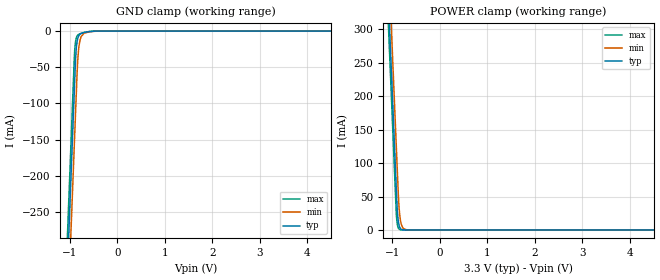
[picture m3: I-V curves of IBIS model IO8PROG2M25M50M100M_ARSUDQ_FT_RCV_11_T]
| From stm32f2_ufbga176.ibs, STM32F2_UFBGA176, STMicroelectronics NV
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| *** New cell (Generated with 5.14beta1 (Sep 20 2010 13:23:23))
[Model]   IO8PROG2M25M50M100M_ARSUDQ_FT_RCV_11_T
Model_type Input
Polarity   Non-Inverting
Enable   Active-Low
| CAP_THRESHOLD on pad IOV33 is "CMOS" :
| Rising=10.0% of vddio   Falling=90.0% of vddio
| C_comp min and max val. don't necessarily correlate with the min and max pvt
| but are the smallest and greatest pad capacitance found.
| var   typ   min   max
C_comp   2.14000pF  2.04120pF  2.26005pF
Vinl = 800.0mV | Dummy value overriden by next lines
Vinh = 2.00V | Dummy value overriden by next lines
[Model Spec]
| TIME_THRESHOLD on pin ZIV33 is "CORE" :
| Rising=40.0% of vddio   Falling=60.0% of vddio
Vinl 1.48450V 1.23350V 1.61250V
Vinh 1.48450V 1.23350V 1.61250V
| variable   typ   min   max
[Temperature Range] 25.0 125.0 -40.0
| variable   typ   min   max
[Voltage Range] 3.3V 2.7V 3.6V
| variable   typ   min   max
[POWER Clamp Reference] 3.3V 2.7V 3.6V
| variable   typ   min   max
[GND Clamp Reference] 0V 0V 0V
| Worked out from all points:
|   GND clamp passes 1 mA (typ) near -0.62 V on its own axis
|   POWER clamp passes 1 mA (typ) near -0.81 V on its own axis
[POWER Clamp]
-3.3V     4.11A      4.173A     4.072A
-1.09V    352.5mA    415.9mA    314.5mA
-1.05V    284.5mA    347.9mA    246.5mA
-1.01V    216.5mA    279.9mA    178.5mA
-920mV    63.51mA    126.9mA    25.85mA
-900mV    31.51mA    92.9mA     9.552mA
-890mV    21.35mA    75.9mA     5.807mA
-870mV    9.804mA    44.01mA    2.146mA
-840mV    3.05mA     18.36mA    482.1uA
-780mV    295.2uA    3.194mA    24.34uA
-660mV    2.764uA    96.54uA    62.42nA
6.6V      0A         0A         0A
[GND Clamp]
-3.3V     -4.149A    -4.223A    -4.103A
-1.06V    -340.6mA   -415.4mA   -294.5mA
-940mV    -136.6mA   -211.4mA   -90.54mA
-900mV    -68.55mA   -143.4mA   -26.55mA
-880mV    -36.73mA   -109.4mA   -13.46mA
-870mV    -26.56mA   -92.4mA    -10.28mA
-840mV    -11.29mA   -44.89mA   -5.954mA
-820mV    -7.224mA   -26.98mA   -4.795mA
-790mV    -4.452mA   -13.31mA   -3.784mA
-700mV    -1.958mA   -2.906mA   -1.882mA
-350mV    -6.427uA   -36.29uA   -1.194uA
6.6V      9.456nA    1.185uA    63.86pA
